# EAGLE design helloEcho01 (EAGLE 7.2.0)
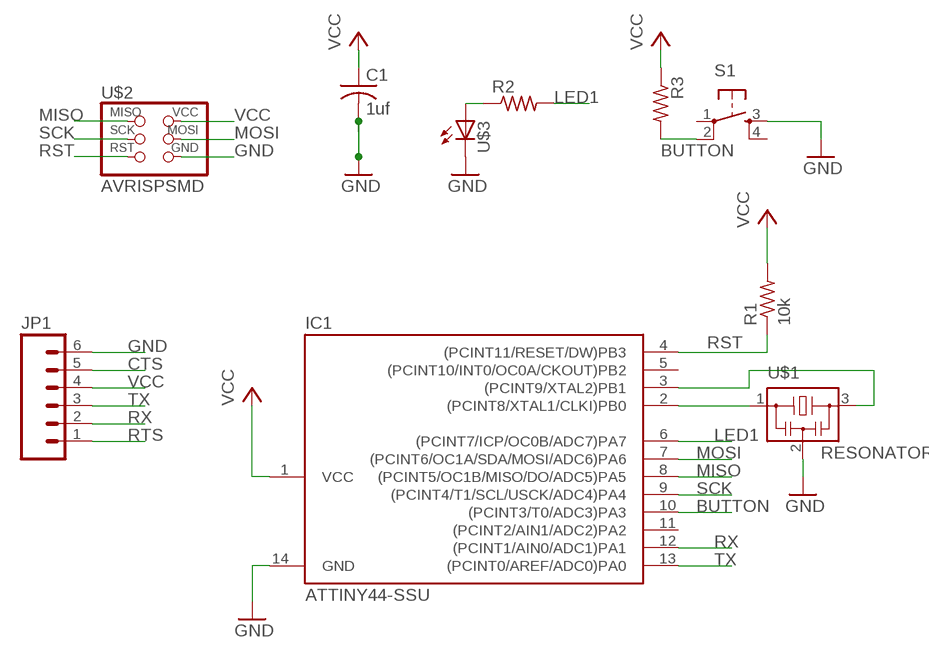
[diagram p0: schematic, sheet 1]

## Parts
C1  1uf  C-USC1206  [C1206]
IC1  ATTINY44-SSU  [SOIC14]
JP1  M06SMD  [1X06-SMD]
R1  10k  R-US_R1206  [R1206]
R2  RESISTOR1206  [1206]
R3  RESISTOR1206  [1206]
S1  6MM_SWITCH6MM_SWITCH  [6MM_SWITCH]
U$1  RESONATOR  [EFOBM]
U$2  AVRISPSMD  [2X03SMD]
U$3  LED1206  [1206]

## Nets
BUTTON: IC1.10((PCINT3/T0/ADC3)PA3) R3.2 S1.2(P1)
CTS: JP1.5
GND: C1.2 IC1.14(GND) JP1.6 S1.3(S) U$1.2 U$2.6(GND) U$3.2(C)
LED1: IC1.6((PCINT7/ICP/OC0B/ADC7)PA7) R2.2
MISO: IC1.8((PCINT5/OC1B/MISO/DO/ADC5)PA5) U$2.1(MISO)
MOSI: IC1.7((PCINT6/OC1A/SDA/MOSI/ADC6)PA6) U$2.4(MOSI)
N$1: IC1.2((PCINT8/XTAL1/CLKI)PB0) U$1.1
N$2: IC1.3((PCINT9/XTAL2)PB1) U$1.3
N$4: R2.1 U$3.1(A)
RST: IC1.4((PCINT11/RESET/DW)PB3) R1.1 U$2.5(RST)
RTS: JP1.1
RX: IC1.12((PCINT1/AIN0/ADC1)PA1) JP1.2
SCK: IC1.9((PCINT4/T1/SCL/USCK/ADC4)PA4) U$2.3(SCK)
TX: IC1.13((PCINT0/AREF/ADC0)PA0) JP1.3
VCC: C1.1 IC1.1(VCC) JP1.4 R1.2 R3.1 U$2.2(VCC)
Unconnected: IC1.5((PCINT10/INT0/OC0A/CKOUT)PB2) IC1.11((PCINT2/AIN1/ADC2)PA2) S1.1(P) S1.4(S1)

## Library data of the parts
C1 = rcl:C-US: CAPACITOR, American symbol
IC1 = fab:ATTINY44
JP1 = SparkFun:M06: Header 6 Standard 6-pin 0.1" header. Use with straight break away headers (SKU : PRT-00116), right angle break away headers (PRT-00553), swiss pins (PRT-00743), machine pins (PRT-00117), and female headers (PRT-00115). Molex polarized connector foot print use with SKU : PRT-08094 with associated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
R1 = resistor:R-US_: RESISTOR, American symbol
R2 R3 = 01_FAB_Hello:RESISTOR
S1 = 01_FAB_Hello:6MM_SWITCH: OMRON SWITCH
U$1 = fab:RESONATOR
U$2 = fab:AVRISP
U$3 = 01_FAB_Hello:LED

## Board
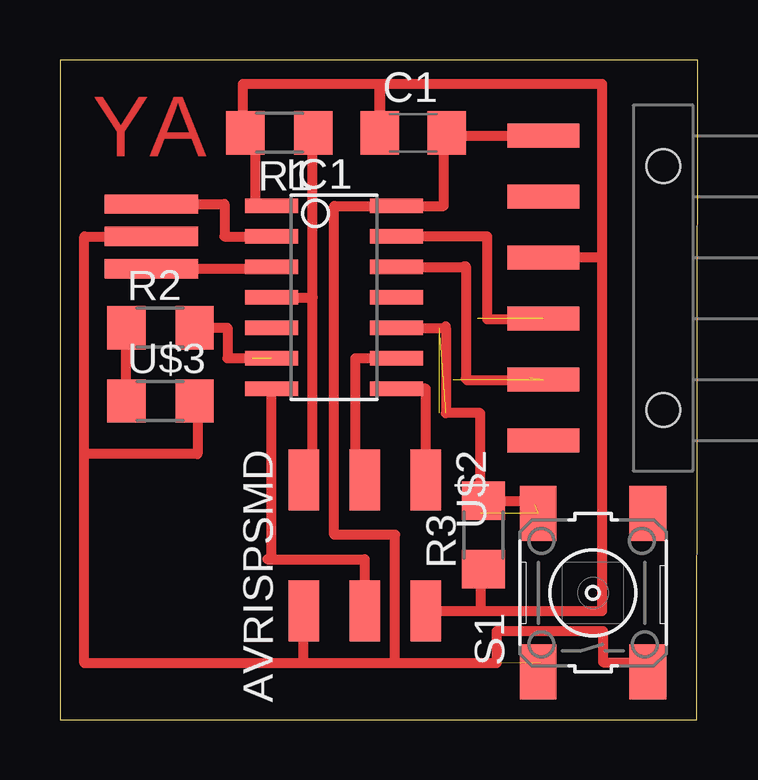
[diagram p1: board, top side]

Size 26.59 x 27.51 mm. Coordinates in mm from the lower left corner, seen from the top.
Outline: 0,0 26.55,0 26.59,27.51 0,27.51 0,0
Copper layers 1: Top 0.035mm
Design rules "ERP-1sided-10mil-16mill": minimum track width 10mil, minimum drill 24mil, track to track 16mil, track to pad 16mil, pad to pad 16mil, via to via 16mil, smd to smd 0mil, copper to edge 16mil, drill to drill 36mil, minimum pad ring 10mil, minimum via ring 8mil, stop-mask expansion 4mil, vias tented up to drill 0mil, thermal gap 10mil

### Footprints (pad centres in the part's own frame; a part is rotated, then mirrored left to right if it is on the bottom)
C1206 = smd 1.6 x 1.8: 1 -1.4,0; 2 1.4,0
SOIC14 = smd 0.61 x 2.21: 1 -3.81,-2.603; 2 -2.54,-2.603; 3 -1.27,-2.603; 4 0,-2.603; 5 1.27,-2.603; 6 2.54,-2.603; 7 3.81,-2.603; 8 3.81,2.603; 9 2.54,2.603; 10 1.27,2.603; 11 0,2.603; 12 -1.27,2.603; 13 -2.54,2.603; 14 -3.81,2.603
1X06-SMD = smd 1 x 3: 1 -6.35,5; 2 -3.81,5; 3 -1.27,5; 4 1.27,5; 5 3.81,5; 6 6.35,5 | hole 1.4: -5.08,0; 5.08,0
R1206 = smd 1.6 x 1.803: 1 -1.422,0; 2 1.422,0
1206 = smd 1.6 x 1.803: 1 -1.422,0; 2 1.422,0
6MM_SWITCH = smd 2.286 x 1.524: 1 -3.302,2.286; 2 3.302,2.286; 3 -3.302,-2.286; 4 3.302,-2.286
EFOBM = smd 0.8 x 3.9: 1 -1.35,0; 2 0,0; 3 1.35,0
2X03SMD = smd 2.54 x 1.27: 1 -2.54,2.54; 2 2.92,2.54; 3 -2.54,0; 4 2.92,0; 5 -2.54,-2.54; 6 2.92,-2.54

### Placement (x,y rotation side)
C1  14.73,24.47 0 top
IC1  11.43,17.61 270 top
JP1  25.15,18 90 top
R1  9.14,24.47 180 top
R2  4.19,16.34 0 top
R3  17.65,7.71 90 top
S1  22.23,5.3 90 top
U$1  3.81,20.15 270 top
U$2  12.7,7.45 270 top
U$3  4.19,13.3 0 top

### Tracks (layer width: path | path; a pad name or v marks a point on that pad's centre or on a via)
BUTTON  (5 unrouted)
  Top 0.406: R3.2 19.81,9.13 19.81,8.98 | 17.53,8.6 17.53,12.79 16.09,12.79 16.09,16.34 | IC1.10 16.09,16.34 | 16.09,16.34 16.09,16.41
GND  (1 unrouted)
  Top 0.406: 13.97,2.37 13.97,7.71 11.43,7.71 11.43,21.42 IC1.14 16,21.42 16,24.47 C1.2 16.13,24.35 JP1.6 20.15,24.6 | 10.16,2.37 13.97,2.37 | U$1.2 1.02,20.15 1.02,11.08 | 1.02,11.08 1.02,2.37 10.16,2.37 | 10.16,2.37 U$2.6 | 20.05,2.39 20.05,2.37 | U$3.2 5.74,13.3 5.74,11.08 1.02,11.08 | 13.97,2.37 18.21,2.37 18.21,3.7 22.64,3.7 22.64,2.41 24.51,2.41 S1.3
LED1  (1 unrouted)
  Top 0.406: R2.2 6.99,16.34 6.99,15.07 8,15.07
MISO
  Top 0.406: IC1.8 15.24,13.8 U$2.1
MOSI
  Top 0.406: 8.64,13.8 IC1.7 8.83,6.69 | 8.83,6.69 12.7,6.69 U$2.4 | 8.64,6.69 8.83,6.69
N$1
  Top 0.406: U$1.1 6.86,21.5 6.86,20.15 IC1.2
N$2
  Top 0.406: U$1.3 8.83,18.8 IC1.3
N$4
  Top 0.406: U$3.1 R2.1
RST
  Top 0.406: R1.1 10.54,24.47 10.54,17.61 | IC1.4 10.54,17.61 | U$2.5 10.54,9.99 10.54,17.61
RX  (2 unrouted)
  Top 0.406: IC1.12 16.86,18.88 16.86,18.9 16.92,18.9 16.92,14.22 16.98,14.22 16.98,14.16 19.58,14.16 19.58,14.28
SCK
  Top 0.406: U$2.3 12.32,9.99 12.32,15.07 IC1.9
TX  (2 unrouted)
  Top 0.406: IC1.13 17.8,20.15 17.8,16.71 19.52,16.71 19.52,16.77
VCC
  Top 0.254: 22.61,5.68 22.61,5.78
  Top 0.406: 22.61,19.27 JP1.4 | 22.61,19.27 22.61,5.68 22.61,4.53 17.53,4.53 | IC1.1 8.13,21.42 8.13,24.47 R1.2 7.62,24.47 7.62,26.5 13.33,26.5 C1.1 13.34,26.5 22.61,26.5 22.61,19.27 | U$2.2 17.53,4.53 | R3.1 17.53,6.29 17.53,4.53

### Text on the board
Top: YA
